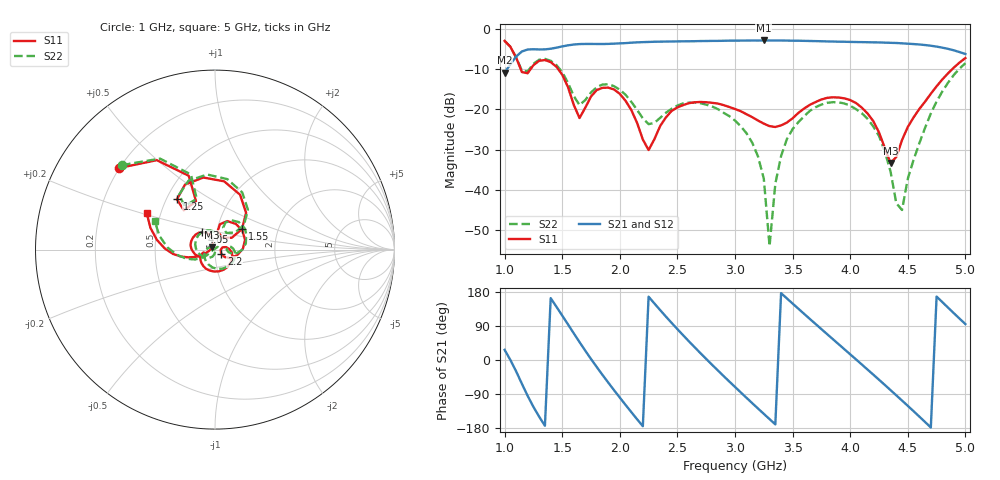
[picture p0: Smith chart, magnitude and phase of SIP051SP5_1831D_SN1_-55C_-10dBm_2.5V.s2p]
# GHz  S  dB  R  50
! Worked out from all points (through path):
!   81 points, 1 GHz to 5 GHz, reference 50 ohm
!   highest |S21| = -2.96 dB at 3.25 GHz (marker M1); lowest = -10.9 dB at 1 GHz (marker M2)
!   lowest |S11| = -33.3 dB at 4.35 GHz (marker M3), VSWR 1.04, Z = 48.3 + j1.29 ohm
!   |S11| at or under -10 dB: 1.139 GHz to 1.227 GHz (87.92 MHz wide, 7.43 % of centre); 1.464 GHz to 4.888 GHz (3.425 GHz wide, 108 % of centre)
!   |S22| runs from -53.9 to -3.1 dB; largest |S21 - S12| = 0.0022
!   S11 on the Smith chart (normalised r, x): 1 GHz: 0.20, +0.35; 1.25 GHz: 0.57, +0.36; 1.55 GHz: 1.31, +0.31; 2.2 GHz: 1.07, -0.05; 4.05 GHz: 0.85, +0.17; 5 GHz: 0.42, +0.21
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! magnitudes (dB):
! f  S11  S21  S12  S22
! 1 GHz  -3.1  -10.9  -10.9  -3.1
! 1.15 GHz  -10.8  -5.7  -5.7  -10.4
! 1.25 GHz  -9.1  -5.1  -5.1  -8.7
! 1.55 GHz  -14.5  -4.2  -4.2  -13.4
! 1.65 GHz  -22.2  -3.9  -3.9  -19.0
! 1.7 GHz  -19.6  -3.8  -3.8  -17.7
! 1.95 GHz  -15.1  -3.7  -3.8  -14.3
! 2.2 GHz  -27.5  -3.4  -3.4  -22.2
! 2.25 GHz  -30.1  -3.3  -3.3  -23.7
! 2.35 GHz  -24.2  -3.3  -3.2  -22.1
! 2.65 GHz  -18.3  -3.1  -3.1  -18.3
! 3 GHz  -19.9  -3.0  -3.0  -22.8
! 3.25 GHz  -23.6  -3.0  -3.0  -37.2
! 3.3 GHz  -24.2  -3.0  -3.0  -53.9
! 3.35 GHz  -24.4  -3.0  -3.0  -38.5
! 3.4 GHz  -24.0  -3.0  -3.0  -31.6
! 3.7 GHz  -18.2  -3.1  -3.1  -19.5
! 4.05 GHz  -18.4  -3.3  -3.3  -20.0
! 4.35 GHz  -33.3  -3.5  -3.6  -35.4
! 4.45 GHz  -27.6  -3.7  -3.7  -44.9
! 4.7 GHz  -16.1  -4.3  -4.3  -21.1
! 5 GHz  -7.3  -6.3  -6.3  -8.6
